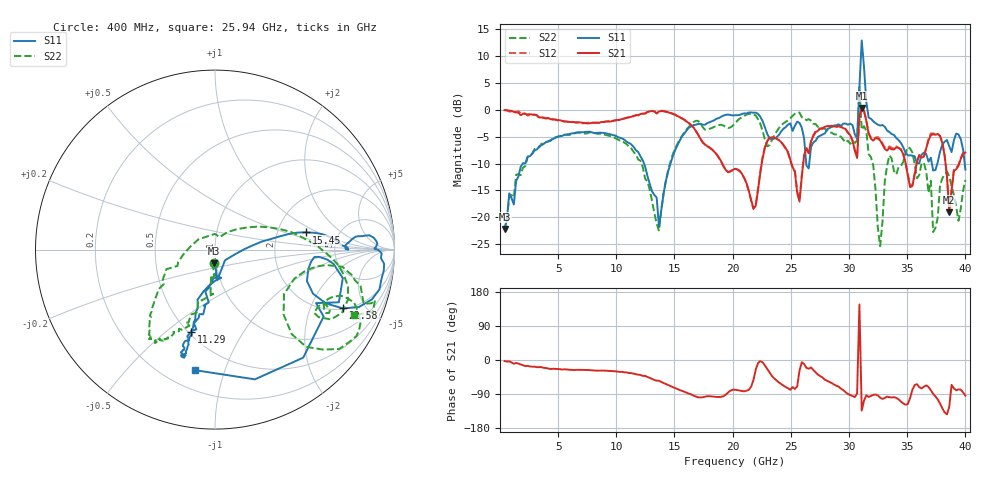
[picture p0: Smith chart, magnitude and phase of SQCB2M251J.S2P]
! Network Analyzer HP8722ES.07.66: Jul 25, 2000 Serial No. US39175408
! 27 Oct 2004  13:39:31
! Frequency  S11  S21  S12  S22
# HZ  S  DB R  50
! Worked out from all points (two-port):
!   201 points, 400 MHz to 40 GHz, reference 50 ohm
!   highest |S21| = 0.34 dB at 31.09 GHz (marker M1); lowest = -19.1 dB at 38.61 GHz (marker M2)
!   |S21| within 3 dB of the highest: start of sweep to 16.35 GHz; 30.85 GHz to 31.54 GHz (685.7 MHz wide, 2.2 % of centre)
!   lowest |S11| = -22.2 dB at 400 MHz (marker M3), VSWR 1.17, Z = 48.6 - j7.55 ohm
!   |S11| at or under -10 dB: start of sweep to 1.959 GHz; 12.38 GHz to 14.65 GHz (2.273 GHz wide, 16.8 % of centre); 26.32 GHz to 26.58 GHz (257.3 MHz wide, 0.973 % of centre)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
!   |S22| runs from -25.4 to 4.3 dB; largest |S21 - S12| = 0.09
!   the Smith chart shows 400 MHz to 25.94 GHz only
!   S11 on the Smith chart (normalised r, x): 400 MHz: 0.97, -0.15; 11.29 GHz: 0.52, -0.61; 15.45 GHz: 2.91, +0.76; 22.58 GHz: 2.03, -3.46; 25.94 GHz: 0.32, -0.79
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4e8  -22.20 -96.1  -0.04 -2.7  0.00 -2.2  -22.43 -93.3
7.132e9  -4.17 -107.7  -2.41 -25.8  -2.50 -26.9  -4.38 -123.3
1.129e10  -6.44 -106.1  -1.28 -34.6  -1.29 -35.1  -7.19 -140.2
1.3666e10  -21.76 -47.1  -0.29 -54.7  -0.24 -55.1  -22.59 69.1
1.5448e10  -5.75 10.7  -1.35 -79.2  -1.35 -80.2  -5.48 4.8
2.02e10  -0.99 0.2  -10.96 -78.6  -10.97 -78.7  -2.52 -20.1
2.2576e10  -2.10 -24.6  -8.98 -6.0  -8.71 -7.1  -3.93 -47.8
2.5348e10  -2.96 -31.6  -11.56 -76.4  -11.27 -79.8  -0.72 -19.0
2.5942e10  -3.34 -99.6  -12.38 -5.9  -12.16 -4.7  -1.36 -25.2
2.6932e10  -6.07 165.9  -4.87 -26.2  -4.70 -28.2  -2.58 -40.2
2.8714e10  -2.89 83.3  -3.10 -64.9  -2.90 -66.1  -4.54 -48.5
3.0694e10  -5.37 29.0  -8.97 -88.0  -8.71 -87.0  -5.69 -96.7
3.0892e10  4.15 -2.3  -1.05 146.5  -1.95 148.2  4.30 8.7
3.109e10  12.95 -61.3  0.34 -133.3  0.22 -132.6  -3.69 149.8
3.1288e10  7.98 -79.9  -0.14 -107.4  -0.22 -106.3  -3.04 -157.0
3.1486e10  1.47 -69.5  -2.04 -93.1  -1.94 -93.0  -3.89 -137.7
3.2674e10  -2.92 -108.3  -5.69 -99.3  -5.45 -101.0  -25.40 53.4
3.3466e10  -4.13 -145.8  -7.11 -98.2  -6.80 -97.9  -8.48 -178.0
3.703e10  -8.90 82.7  -4.71 -79.7  -4.39 -79.9  -13.20 50.2
3.7228e10  -11.29 63.5  -4.54 -89.5  -4.38 -89.8  -22.77 127.2
3.8614e10  -6.77 -90.0  -19.06 -123.5  -18.88 -123.3  -12.32 93.6
4e10  -11.12 179.5  -7.92 -93.9  -7.81 -94.2  -13.06 -142.7
